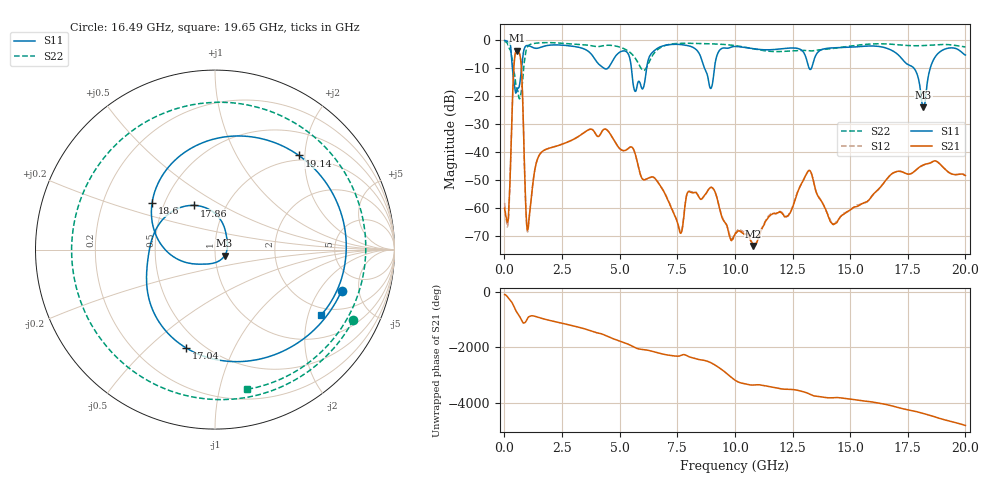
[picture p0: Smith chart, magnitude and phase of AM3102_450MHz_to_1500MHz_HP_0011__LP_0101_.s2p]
!Agilent Technologies,E8364B,MY43040894,A.07.50.67
!Agilent E8364B: A.07.50.67
!Date: Thursday, January 11, 2018 05:31:21
!Correction: S11(Full 2 Port(1,2))
!S21(Full 2 Port(1,2))
!S12(Full 2 Port(1,2))
!S22(Full 2 Port(1,2))
!S2P File: Measurements: S11, S21, S12, S22:
# Hz S  dB  R 50
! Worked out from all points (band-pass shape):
!   1601 points, 10 MHz to 20 GHz, reference 50 ohm
!   highest |S21| = -3.66 dB at 547.2 MHz (marker M1); lowest = -73.6 dB at 10.79 GHz (marker M2)
!   |S21| within 3 dB of the highest: 440.5 MHz to 702.4 MHz (261.9 MHz wide, 45.8 % of centre)
!   lowest |S11| = -24.0 dB at 18.18 GHz (marker M3), VSWR 1.14, Z = 55.5 - j3.85 ohm
!   |S11| at or under -10 dB: 5.511 GHz to 6.171 GHz (660.1 MHz wide, 11.3 % of centre); 8.683 GHz to 9.111 GHz (427.9 MHz wide, 4.81 % of centre); 17.77 GHz to 18.47 GHz (705.4 MHz wide, 3.89 % of centre)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
!   |S22| runs from -21.0 to -0.4 dB; largest |S21 - S12| = 0.0081
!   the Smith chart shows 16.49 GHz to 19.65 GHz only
!   S11 on the Smith chart (normalised r, x): 16.49 GHz: 3.22, -3.28; 17.04 GHz: 0.41, -0.67; 17.86 GHz: 0.71, +0.38; 18.6 GHz: 0.43, +0.27; 19.14 GHz: 0.91, +1.88; 19.65 GHz: 1.73, -2.43
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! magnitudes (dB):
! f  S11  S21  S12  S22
! 10 MHz  -0.1  -60.1  -58.2  -0.4
! 172.4 MHz  -0.6  -63.7  -64.4  -2.0
! 547.2 MHz  -18.0  -3.7  -3.7  -17.7
! 722.1 MHz  -11.6  -8.1  -8.1  -18.8
! 1.022 GHz  -1.9  -67.7  -68.4  -2.1
! 1.534 GHz  -2.6  -40.8  -40.8  -0.9
! 3.346 GHz  -2.8  -33.7  -33.7  -1.6
! 5.682 GHz  -18.3  -40.8  -40.8  -6.5
! 6.682 GHz  -2.7  -51.1  -51.1  -3.1
! 10.01 GHz  -2.2  -69.4  -69.3  -1.9
! 10.79 GHz  -3.0  -73.6  -73.2  -3.0
! 13.34 GHz  -9.6  -48.2  -48.1  -3.8
! 14.29 GHz  -2.7  -65.9  -65.9  -2.9
! 16.49 GHz  -2.6  -50.7  -50.8  -1.3
! 16.68 GHz  -3.1  -48.8  -48.9  -1.3
! 17.04 GHz  -4.9  -46.9  -47.0  -1.6
! 17.86 GHz  -11.3  -46.4  -46.4  -2.0
! 18.18 GHz  -24.0  -44.6  -44.7  -1.9
! 18.6 GHz  -7.2  -43.3  -43.3  -1.7
! 19.14 GHz  -3.1  -46.3  -46.3  -1.5
! 19.65 GHz  -3.2  -48.1  -48.1  -2.0
! 20 GHz  -5.3  -48.4  -48.2  -2.4
